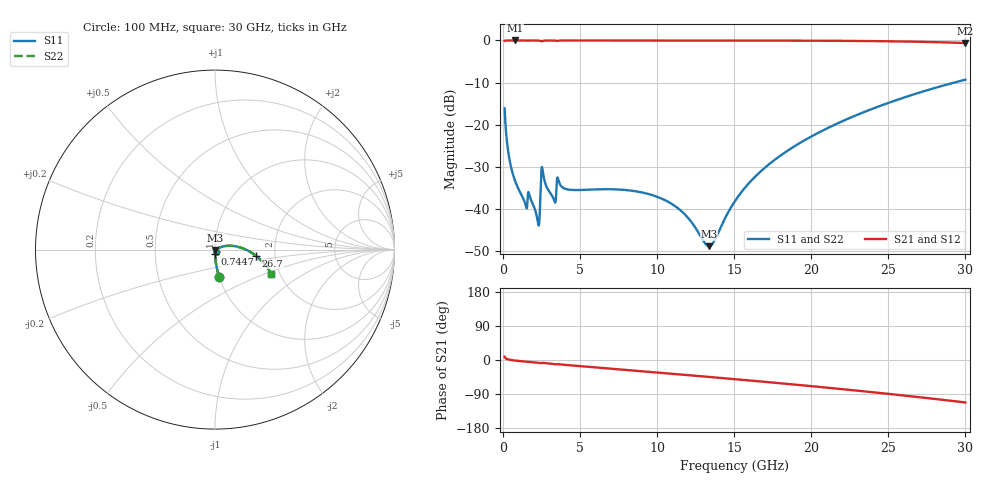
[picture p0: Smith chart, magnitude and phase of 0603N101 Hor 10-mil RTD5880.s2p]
# GHz S MA R 50
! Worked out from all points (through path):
!   3201 points, 100 MHz to 30 GHz, reference 50 ohm
!   highest |S21| = -0.01 dB at 754.1 MHz (marker M1); lowest = -0.6 dB at 30 GHz (marker M2)
!   group delay of S21, straight-line fit = 10.3 ps
!   lowest |S11| = -48.9 dB at 13.37 GHz (marker M3), VSWR 1.01, Z = 50.2 - j0.261 ohm
!   |S11| at or under -10 dB: start of sweep to 29.29 GHz
!   |S22| runs from -48.9 to -9.3 dB; largest |S21 - S12| = 0
!   S11 on the Smith chart (normalised r, x): 100 MHz: 1.00, -0.32; 744.7 MHz: 1.00, -0.04; 26.7 GHz: 1.58, -0.11; 30 GHz: 1.81, -0.55
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0.1  0.1559 -81.3  0.9875 8.6  0.9875 8.6  0.1559 -81.3
0.3896562  0.04107 -88.2  0.9986 1.0  0.9986 1.0  0.04107 -88.2
0.7447187  0.02233 -89.2  0.9989 -1.3  0.9989 -1.3  0.02233 -89.2
0.7540625  0.02208 -89.2  0.9989 -1.3  0.9989 -1.3  0.02208 -89.2
1.426813  0.01168 -86.3  0.9983 -4.2  0.9983 -4.2  0.01168 -86.3
1.763187  0.01344 -85.8  0.9977 -5.3  0.9977 -5.3  0.01344 -85.8
2.230375  0.00738 -72.8  0.9969 -7.3  0.9969 -7.3  0.00738 -72.8
2.305125  0.006327 -51.7  0.9954 -7.7  0.9954 -7.7  0.006327 -51.7
2.510687  0.03111 -43.1  0.9745 -7.6  0.9745 -7.6  0.03111 -43.1
2.594781  0.02669 -74.1  0.9891 -7.5  0.9891 -7.5  0.02669 -74.1
3.286219  0.01302 -86.6  0.9967 -10.6  0.9967 -10.6  0.01302 -86.6
3.622594  0.02089 -89.6  0.9955 -11.3  0.9955 -11.3  0.02089 -89.6
5.089563  0.01673 -99.2  0.9977 -16.5  0.9977 -16.5  0.01673 -99.2
10.06978  0.01372 -110.7  0.9968 -33.3  0.9968 -33.3  0.01372 -110.7
11.68625  0.008972 -107.4  0.9965 -38.8  0.9965 -38.8  0.008972 -107.4
13.36812  0.003595 -46.3  0.9962 -44.7  0.9962 -44.7  0.003595 -46.3
15.05  0.01236 20.8  0.9958 -50.6  0.9958 -50.6  0.01236 20.8
17.05891  0.03152 24.2  0.9949 -57.9  0.9949 -57.9  0.03152 24.2
20.03956  0.07286 16.9  0.992 -69.1  0.992 -69.1  0.07286 16.9
25.01978  0.1815 -1.4  0.9767 -89.4  0.9767 -89.4  0.1815 -1.4
26.70166  0.2302 -8.5  0.966 -96.8  0.966 -96.8  0.2302 -8.5
30  0.3419 -23.3  0.9315 -112.0  0.9315 -112.0  0.3419 -23.3
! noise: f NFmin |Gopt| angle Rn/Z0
0.1  0.0002674  0.9112  0.3832  0.0006624
3.417  0.007576  0.8943  11.73  0.01546
6.743  0.00593  0.7556  23.05  0.004712
10.06  0.008025  0.7377  34.06  0.005608
13.39  0.01007  0.7292  44.74  0.006357
16.7  0.01212  0.7267  54.96  0.006986
20.03  0.01424  0.7285  64.73  0.00752
23.35  0.01647  0.7334  73.99  0.007971
26.67  0.01887  0.7408  82.79  0.00835
30  0.02148  0.75  91.14  0.008662
